FUNCTION_BLOCK Motor_Current_AC_Drives_DUT

VAR_IN_OUT
    SD_SMD_IO: DUT_AMCI_Stepper;
	 	
END_VAR	

VAR_INPUT
	FB_Motor_Current: UINT;
END_VAR

VAR_OUTPUT
	Enable: BOOL;
	Error: BOOL;
END_VAR

VAR	
	I_Command_Word_1: UINT;
		
END_VAR

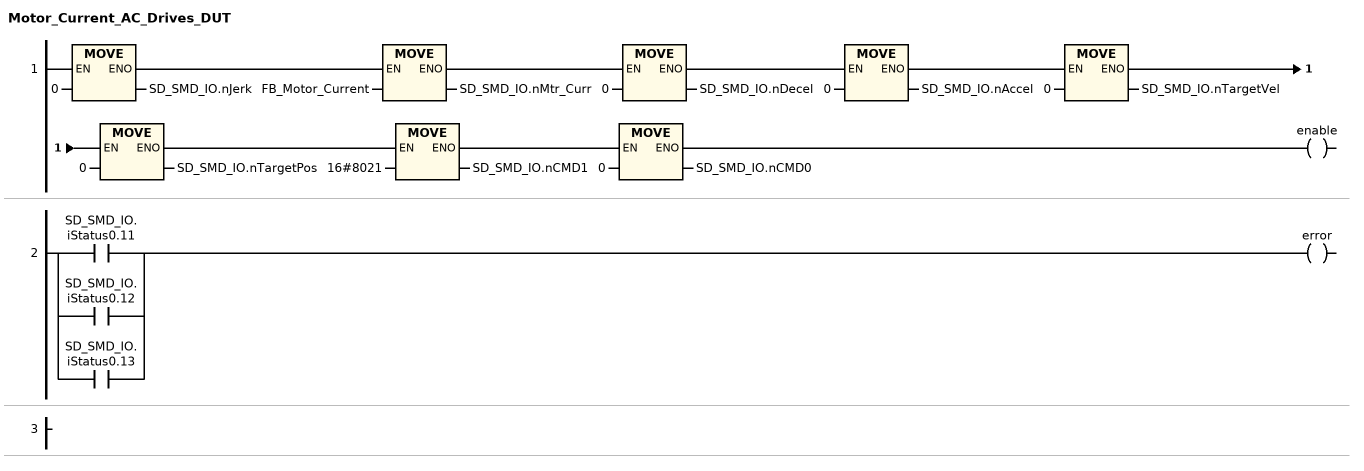
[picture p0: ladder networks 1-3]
// NETWORK 1
SD_SMD_IO.nJerk := 0;
SD_SMD_IO.nMtr_Curr := FB_Motor_Current;
SD_SMD_IO.nDecel := 0;
SD_SMD_IO.nAccel := 0;
SD_SMD_IO.nTargetVel := 0;
SD_SMD_IO.nTargetPos := 0;
SD_SMD_IO.nCMD1 := 16#8021;
SD_SMD_IO.nCMD0 := 0;
enable := TRUE;

// NETWORK 2
error := SD_SMD_IO.iStatus0.11 OR SD_SMD_IO.iStatus0.12 OR SD_SMD_IO.iStatus0.13;

// NETWORK 3

END_FUNCTION_BLOCK
